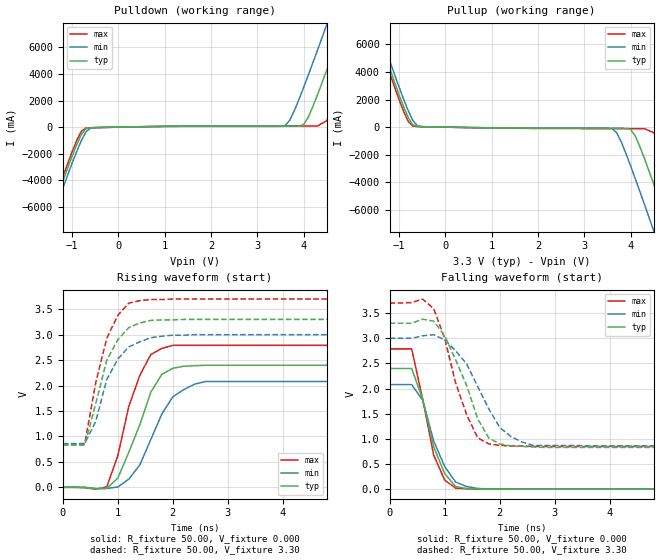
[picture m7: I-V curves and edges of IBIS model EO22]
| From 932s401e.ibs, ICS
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|   Model EO22
[Model]   EO22
Model_type   Output
Polarity   Non-Inverting
C_comp   2.50pF   2.00pF   3.00pF
[Temperature Range]   27.00   70.00   0.000
[Voltage Range]   3.30V   3.00V   3.70V
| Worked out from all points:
|   slope of the pulldown table from 0 to 0.495 V, typ, clamps not added: 15.1 ohm
|   slope of the pullup table from 0 to 0.495 V, typ, clamps not added: 17.1 ohm
|   rising waveform, R_fixture 50.00, V_fixture 0.000: 20-80 % time 511ps typ, 549ps min, 436ps max; typ from 0 V to 2.4 V
|   rising waveform, R_fixture 50.00, V_fixture 3.30: 20-80 % time 433ps typ, 449ps min, 396ps max; typ from 0.83 V to 3.3 V
|   falling waveform, R_fixture 50.00, V_fixture 0.000: 20-80 % time 378ps typ, 396ps min, 337ps max; typ from 2.4 V to 0 V
|   falling waveform, R_fixture 50.00, V_fixture 3.30: 20-80 % time 538ps typ, 632ps min, 470ps max; typ from 3.3 V to 0.83 V
[Pulldown]
| voltage   I(typ)   I(min)   I(max)
-3.3V     -24.56A    -25.06A    -24.24A
-1.7V     -8.82A     -9.35A     -8.5A
-1.5V     -6.89A     -7.42A     -6.56A
-900mV    -1.32A     -1.84A     -1.01A
-700mV    -110mA     -360mA     -63.12mA
3.6V      73.9mA     120mA      91.09mA
4V        200mA      3A         91.37mA
4.3V      2.45A      5.81A      92.16mA
4.5V      4.31A      7.73A      490mA
4.9V      8.15A      11.62A     3.97A
5.3V      12.06A     15.54A     7.82A
6.6V      24.92A     28.41A     20.63A
[Pullup]
| voltage   I(typ)   I(min)   I(max)
-3.3V     24.76A     25.29A     24.43A
-1.7V     9.02A      9.58A      8.68A
-1.5V     7.09A      7.65A      6.74A
-900mV    1.5A       2.04A      1.16A
-700mV    160mA      490mA      73.7mA
-500mV    33.32mA    32.07mA    36.49mA
3.6V      -85.84mA   -100mA     -110mA
4V        -160mA     -2.8A      -110mA
4.5V      -4.13A     -7.52A     -400mA
4.9V      -7.98A     -11.42A    -3.82A
5.3V      -11.9A     -15.35A    -7.67A
6.6V      -24.77A    -28.24A    -20.51A
[Ramp]
| variable   typ   min   max
dV/dt_r   1.44/0.45n   1.25/0.53n   1.67/0.37n
dV/dt_f   1.48/0.46n   1.28/0.60n   1.71/0.39n
R_load = 50.00
[Rising Waveform]
R_fixture = 50.00
V_fixture = 0.000
V_fixture_min = 0.000
V_fixture_max = 0.000
| time   V(typ)   V(min)   V(max)
0s        0V         0V         0V
800ps     -20.98mV   -21.72mV   10.79mV
1ns       180mV      6.24mV     620mV
1.2ns     690mV      160mV      1.59V
1.4ns     1.23V      440mV      2.2V
1.6ns     1.87V      940mV      2.61V
1.8ns     2.22V      1.44V      2.73V
2ns       2.34V      1.78V      2.79V
2.6ns     2.4V       2.08V      2.79V
10ns      2.4V       2.08V      2.79V
[Rising Waveform]
R_fixture = 50.00
V_fixture = 3.30
V_fixture_min = 3.00
V_fixture_max = 3.70
| time   V(typ)   V(min)   V(max)
0s        830mV      860mV      850mV
400ps     830mV      860mV      860mV
600ps     1.65V      1.3V       2.06V
800ps     2.5V       2.12V      2.93V
1ns       2.9V       2.52V      3.38V
1.2ns     3.14V      2.76V      3.62V
1.4ns     3.23V      2.86V      3.67V
1.6ns     3.28V      2.94V      3.69V
2ns       3.29V      2.99V      3.7V
10ns      3.3V       3V         3.7V
[Falling Waveform]
R_fixture = 50.00
V_fixture = 0.000
V_fixture_min = 0.000
V_fixture_max = 0.000
| time   V(typ)   V(min)   V(max)
0s        2.4V       2.08V      2.79V
400ps     2.4V       2.08V      2.79V
600ps     1.79V      1.77V      1.79V
800ps     840mV      960mV      680mV
1ns       310mV      450mV      180mV
1.2ns     50.54mV    140mV      18.99mV
1.4ns     12mV       52.35mV    8.55mV
1.6ns     4.06mV     13.94mV    670uV
2ns       1.3mV      1.01mV     1.67mV
10ns      17.46uV    0V         -4.09uV
[Falling Waveform]
R_fixture = 50.00
V_fixture = 3.30
V_fixture_min = 3.00
V_fixture_max = 3.70
| time   V(typ)   V(min)   V(max)
0s        3.3V       3V         3.7V
600ps     3.38V      3.05V      3.78V
800ps     3.34V      3.07V      3.59V
1ns       3.05V      2.97V      3V
1.4ns     2.06V      2.49V      1.48V
1.6ns     1.4V       2.04V      1.02V
1.8ns     1.02V      1.6V       900mV
2ns       900mV      1.23V      870mV
2.6ns     840mV      870mV      850mV
10ns      830mV      860mV      850mV
